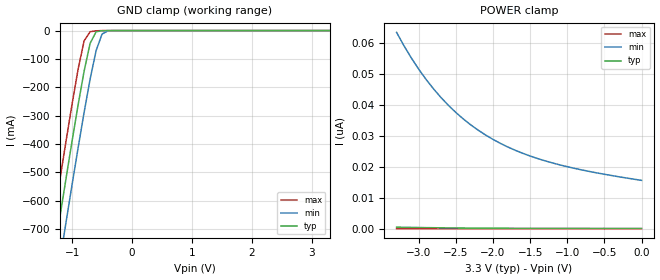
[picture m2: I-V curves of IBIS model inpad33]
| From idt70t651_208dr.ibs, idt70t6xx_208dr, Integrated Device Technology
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|   Model inpad33
[Model]   inpad33
Model_type   Input
Polarity   Non-Inverting
Vinl =  0.80000V
Vinh =  2.00000V
Vmeas =  1.50000V
C_comp   4.50000pF   4.50000pF   4.50000pF
[Temperature Range]   25.00000   100.00000   -40.00000
[Voltage Range]   3.30000V   3.10000V   3.50000V
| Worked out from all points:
|   GND clamp passes 1 mA (typ) near -0.52 V on its own axis
[GND_clamp]
| voltage   I(typ)   I(min)   I(max)
-3.3V     -3.553A    -3.699A    -3.43A
-1.4V     -921.5mA   -1.075A    -790.4mA
-1.3V     -786.2mA   -940.4mA   -654.7mA
-1.2V     -651.9mA   -806.3mA   -520.2mA
-1.1V     -519.1mA   -673.5mA   -387.5mA
-900mV    -262mA     -413.5mA   -136.1mA
-800mV    -143.3mA   -288.9mA   -36.33mA
-700mV    -45.49mA   -171.6mA   -3.972mA
-600mV    -4.309mA   -71.06mA   -834.5uA
-500mV    -411.8uA   -12.18mA   -82.9uA
-400mV    -35.7uA    -828.2uA   -3.321uA
3.3V      60.32pA    16.33nA    261.7fA
[POWER_clamp]
| voltage   I(typ)   I(min)   I(max)
-3.3V     485.3pA    63.31nA    1.192pA
-3.2V     440.5pA    58.98nA    1.104pA
-3V       362.8pA    51.38nA    959fA
-2.9V     329.2pA    48.06nA    890.9fA
-2.7V     271.6pA    42.26nA    779.3fA
-2.4V     205pA      35.37nA    648fA
-2.1V     157.4pA    30.2nA     551.4fA
-1.9V     133.8pA    27.5nA     498.7fA
-1.7V     115.4pA    25.27nA    457.1fA
-1.3V     90.21pA    21.88nA    391.5fA
-700mV    70.52pA    18.44nA    327.3fA
0V        60.32pA    15.58nA    275.6fA
